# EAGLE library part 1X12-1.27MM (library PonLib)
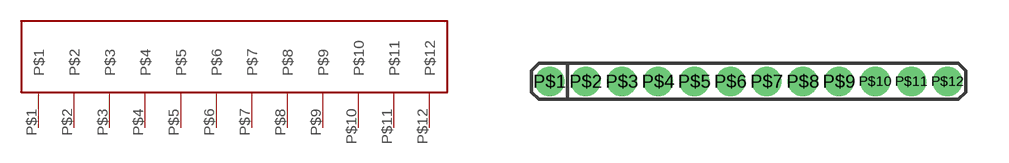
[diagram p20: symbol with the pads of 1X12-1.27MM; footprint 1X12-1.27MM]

Designator prefix -

## 1X12-1.27MM  [1X12-1.27MM]
P$1  P$1
P$2  P$2
P$3  P$3
P$4  P$4
P$5  P$5
P$6  P$6
P$7  P$7
P$8  P$8
P$9  P$9
P$10  P$10
P$11  P$11
P$12  P$12

## Footprint 1X12-1.27MM (pad centres in mm)
drill 0.533 pad 0.889: P$1 -6.985,0; P$2 -5.715,0; P$3 -4.445,0; P$4 -3.175,0; P$5 -1.905,0; P$6 -0.635,0; P$7 0.635,0; P$8 1.905,0; P$9 3.175,0; P$10 4.445,0; P$11 5.715,0; P$12 6.985,0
